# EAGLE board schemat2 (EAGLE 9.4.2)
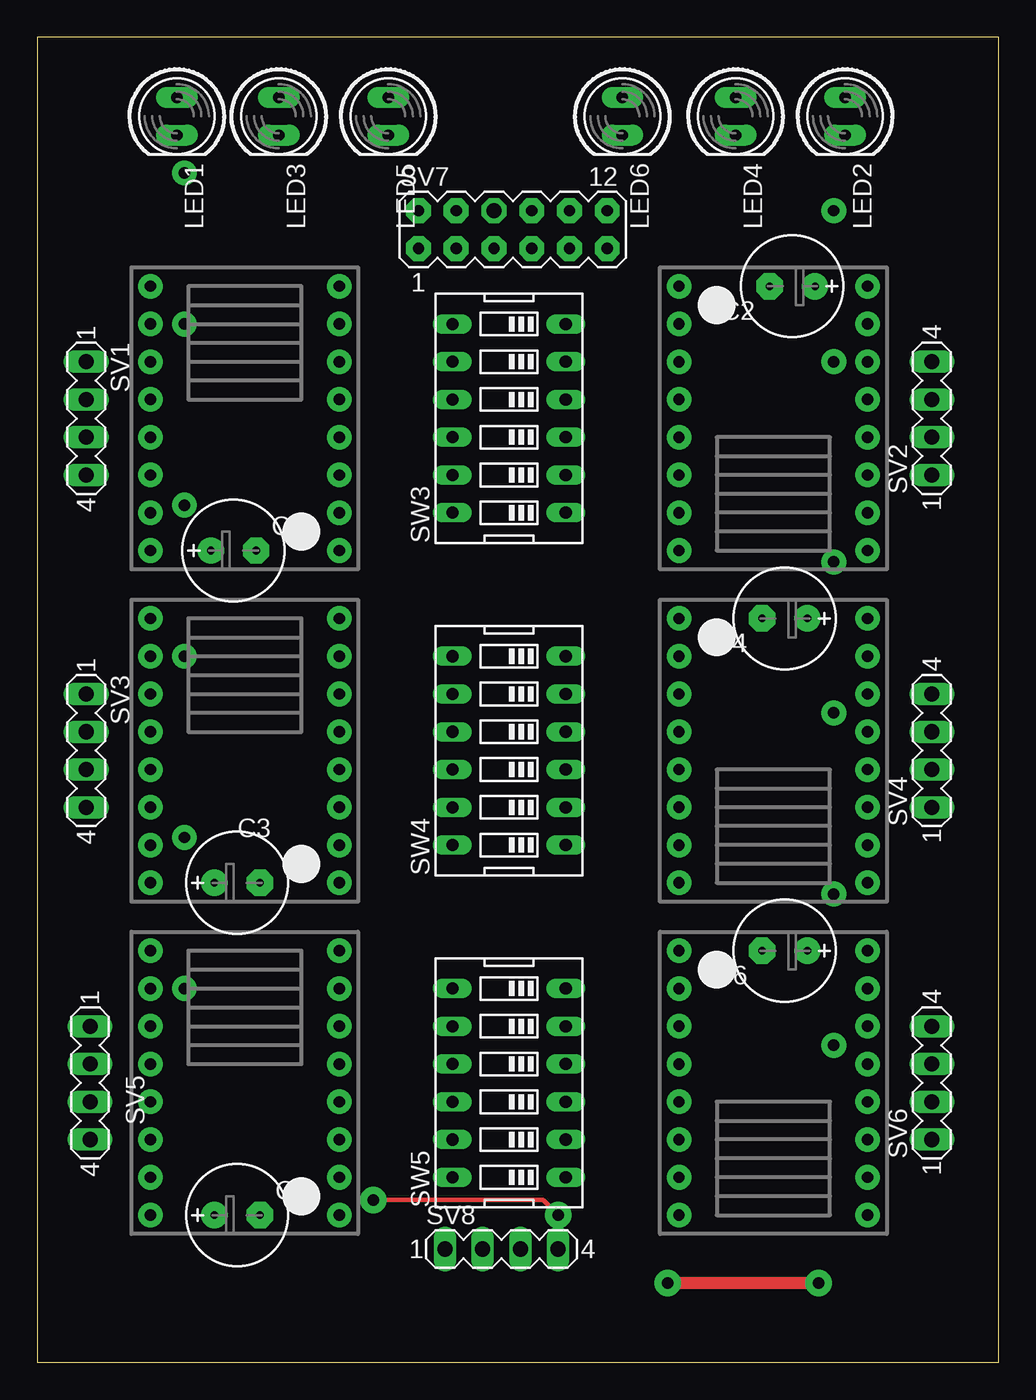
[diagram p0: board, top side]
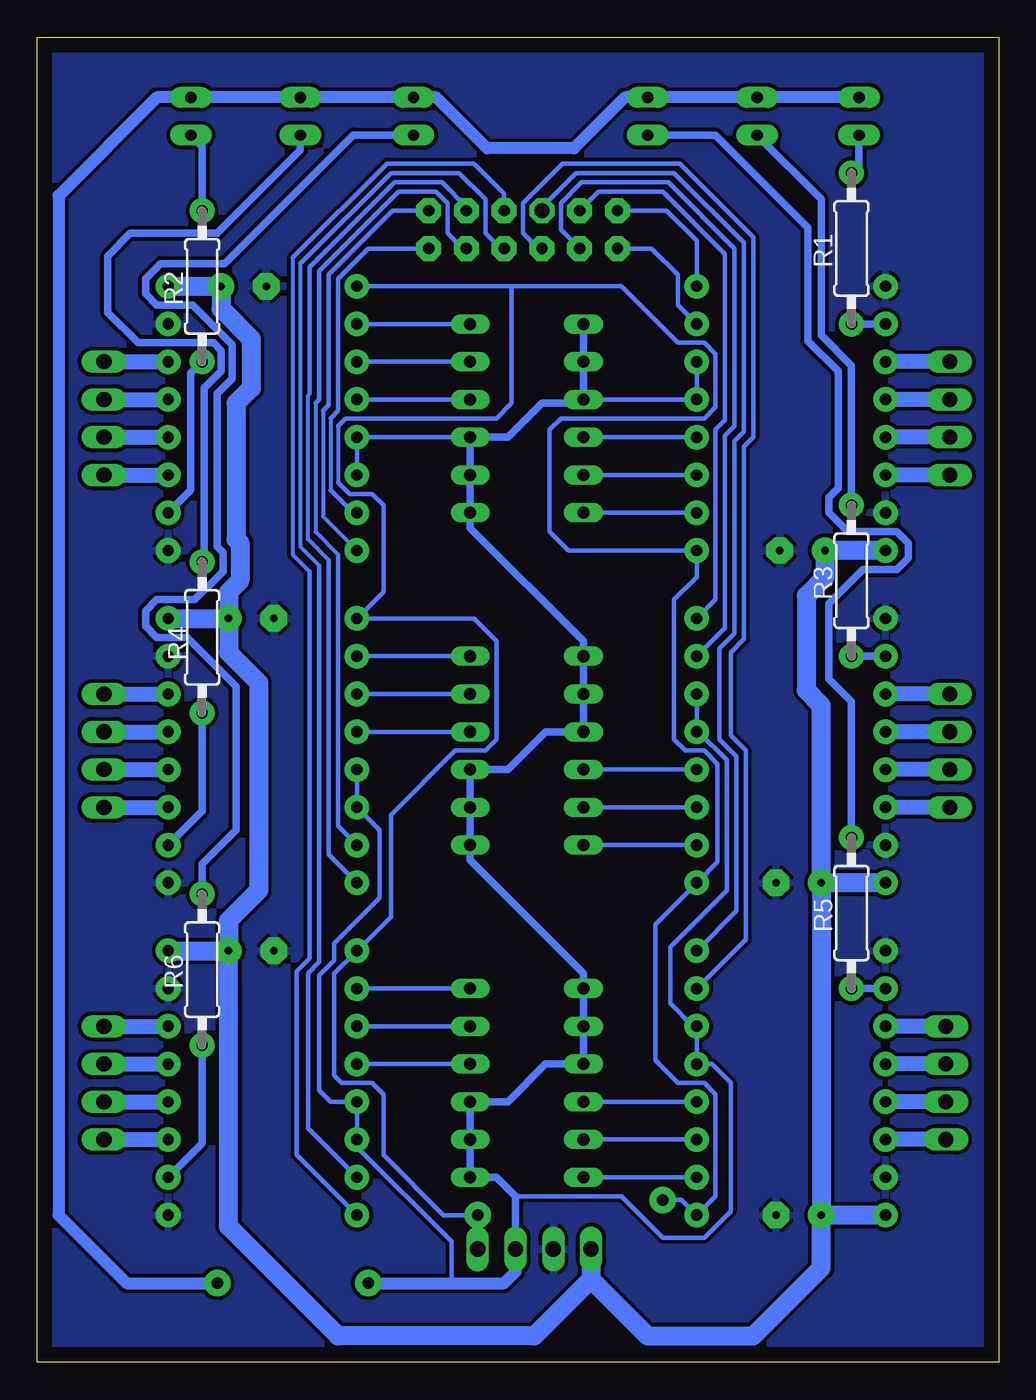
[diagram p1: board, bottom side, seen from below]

Size 64.69 x 89.14 mm. Coordinates in mm from the lower left corner, seen from the top.
Outline: 0,0 64.69,0 64.69,89.14 0,89.14 0,0
Copper layers (1*16): Top 0.035mm / dielectric 1.5mm / Bottom 0.035mm
Design rules "default *": minimum track width 6mil, minimum drill 0.35mm, track to track 8mil, track to pad 8mil, pad to pad 10mil, via to via 10mil, smd to smd 6mil, copper to edge 40mil, drill to drill 6mil, minimum pad ring 10mil, minimum via ring 8mil, stop-mask expansion 4mil, vias tented up to drill 0mil, thermal gap 10mil

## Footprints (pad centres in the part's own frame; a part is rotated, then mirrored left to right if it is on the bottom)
E2,5-7 = drill 0.508 pad 1.778: + -1.524,0 | drill 0.508 pad 1.778 octagon: - 1.524,0
LED5MM = drill 0.762 pad 1.397 long: A -1.27,0; K 1.27,0
0207/10 = drill 0.762 pad 1.676: 1 -5.08,0; 2 5.08,0
MA04-1 = drill 1.016 long: 1 -3.81,0; 2 -1.27,0; 3 1.27,0; 4 3.81,0
MA06-2 = drill 0.762 pad 1.676 octagon: 1 -6.35,-1.27; 2 -6.35,1.27; 3 -3.81,-1.27; 4 -3.81,1.27; 5 -1.27,-1.27; 7 1.27,-1.27; 8 1.27,1.27; 9 3.81,-1.27; 10 3.81,1.27; 11 6.35,-1.27; 12 6.35,1.27 | drill 1.016 pad 1.676 octagon: 6 -1.27,1.27
EDG-06 = drill 0.813 long: 1 -6.35,-3.81; 2 -3.81,-3.81; 3 -1.27,-3.81; 4 1.27,-3.81; 5 3.81,-3.81; 6 6.35,-3.81; 7 6.35,3.81; 8 3.81,3.81; 9 1.27,3.81; 10 -1.27,3.81; 11 -3.81,3.81; 12 -6.35,3.81
DRV8825 = drill 0.762 pad 1.651: 1 -6.35,8.89; 2 -6.35,6.35; 3 -6.35,3.81; 4 -6.35,1.27; 5 -6.35,-1.27; 6 -6.35,-3.81; 7 -6.35,-6.35; 8 -6.35,-8.89; 9 6.35,-8.89; 10 6.35,-6.35; 11 6.35,-3.81; 12 6.35,-1.27; 13 6.35,1.27; 14 6.35,3.81; 15 6.35,6.35; 16 6.35,8.89

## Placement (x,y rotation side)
C1  [E2,5-7]  13.21,54.61 0 top
C2  [E2,5-7]  50.8,72.39 180 top
C3  [E2,5-7]  13.46,32.26 0 top
C4  [E2,5-7]  50.29,50.04 180 top
C5  [E2,5-7]  13.46,9.91 0 top
C6  [E2,5-7]  50.29,27.69 180 top
LED1  [LED5MM]  9.4,83.82 270 top
LED2  [LED5MM]  54.36,83.82 270 top
LED3  [LED5MM]  16.26,83.82 270 top
LED4  [LED5MM]  46.99,83.82 270 top
LED5  [LED5MM]  23.62,83.82 270 top
LED6  [LED5MM]  39.37,83.82 270 top
R1  [0207/10]  9.91,74.93 90 bottom
R2  [0207/10]  53.59,72.39 90 bottom
R3  [0207/10]  9.91,52.58 90 bottom
R4  [0207/10]  53.59,48.77 90 bottom
R5  [0207/10]  9.91,30.23 90 bottom
R6  [0207/10]  53.59,26.42 90 bottom
SV1  [MA04-1]  3.3,63.5 270 top
SV2  [MA04-1]  60.2,63.5 90 top
SV3  [MA04-1]  3.3,41.15 270 top
SV4  [MA04-1]  60.2,41.15 90 top
SV5  [MA04-1]  3.56,18.8 270 top
SV6  [MA04-1]  60.2,18.8 90 top
SV7  [MA06-2]  32,76.2 0 top
SV8  [MA04-1]  31.24,7.62 0 top
SW3  [EDG-06]  31.75,63.5 90 top
SW4  [EDG-06]  31.75,41.15 90 top
SW5  [EDG-06]  31.75,18.8 90 top
U$1  DRV8825  [DRV8825]  13.97,63.5 180 top
U$2  DRV8825  [DRV8825]  49.53,63.5 0 top
U$3  DRV8825  [DRV8825]  13.97,41.15 180 top
U$4  DRV8825  [DRV8825]  49.53,41.15 0 top
U$5  DRV8825  [DRV8825]  13.97,18.8 180 top
U$6  DRV8825  [DRV8825]  49.53,18.8 0 top

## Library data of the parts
C1-C6 = my-rcl; SPICEPREFIX: C
LED1-LED6 = myled
R1-R6 = rcl2; SPICEPREFIX: R
SV1-SV6 SV8 = con-lstb; OC_FARNELL: unknown; OC_NEWARK: unknown
SV7 = my-con-lstb; OC_FARNELL: unknown; OC_NEWARK: unknown
SW3-SW5 = special
U$1-U$6 = robot-driver

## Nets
AX1_DIR: SV7.2 U$1.8
AX1_FLT: R1.1 U$1.10
AX1_M0: SW3.12 U$1.2
AX1_M1: SW3.11 U$1.3
AX1_M2: SW3.10 U$1.4
AX1_STEP: SV7.1 U$1.7
AX2_DIR: SV7.12 U$2.8
AX2_FLT: R2.1 U$2.10
AX2_M0: SW3.6 U$2.2
AX2_M1: SW3.5 U$2.3
AX2_M2: SW3.4 U$2.4
AX2_STEP: SV7.11 U$2.7
AX3_DIR: SV7.4 U$3.8
AX3_FLT: R3.1 U$3.10
AX3_M0: SW4.12 U$3.2
AX3_M1: SW4.11 U$3.3
AX3_M2: SW4.10 U$3.4
AX3_STEP: SV7.3 U$3.7
AX4_DIR: SV7.10 U$4.8
AX4_FLT: R4.1 U$4.10
AX4_M0: SW4.6 U$4.2
AX4_M1: SW4.5 U$4.3
AX4_M2: SW4.4 U$4.4
AX4_STEP: SV7.9 U$4.7
AX5_DIR: SV7.6 U$5.8
AX5_FLT: R5.1 U$5.10
AX5_M0: SW5.12 U$5.2
AX5_M1: SW5.11 U$5.3
AX5_M2: SW5.10 U$5.4
AX5_STEP: SV7.5 U$5.7
AX6_DIR: SV7.8 U$6.8
AX6_FLT: R6.1 U$6.10
AX6_M0: SW5.6 U$6.2
AX6_M1: SW5.5 U$6.3
AX6_M2: SW5.4 U$6.4
AX6_STEP: SV7.7 U$6.7
GND: C1.- C2.- C3.- C4.- C5.- C6.- SV8.2 U$1.9 U$1.15 U$2.9 U$2.15 U$3.9 U$3.15 U$4.9 U$4.15 U$5.9 U$5.15 U$6.9 U$6.15
M_EN: SV8.4 U$1.1 U$2.1 U$3.1 U$4.1 U$5.1 U$6.1
N$1: SV4.1 U$4.11
N$2: LED1.K R1.2
N$3: LED2.K R2.2
N$4: LED3.K R3.2
N$5: LED4.K R4.2
N$6: LED5.K R5.2
N$7: SV4.2 U$4.12
N$8: LED6.K R6.2
N$9: SV5.2 U$5.12
N$10: SV5.1 U$5.11
N$11: SV6.2 U$6.12
N$12: SV6.1 U$6.11
N$13: SV3.2 U$3.12
N$14: SV3.1 U$3.11
N$15: SV2.2 U$2.12
N$16: SV2.1 U$2.11
N$17: SV1.2 U$1.12
N$18: SV1.1 U$1.11
N$21: SV1.4 U$1.14
N$22: SV1.3 U$1.13
N$25: SV2.4 U$2.14
N$26: SV2.3 U$2.13
N$29: SV5.4 U$5.14
N$30: SV5.3 U$5.13
N$33: SV6.4 U$6.14
N$34: SV6.3 U$6.13
N$35: SV4.3 U$4.13
N$36: SV4.4 U$4.14
N$41: SV3.4 U$3.14
N$42: SV3.3 U$3.13
VCC: LED1.A LED2.A LED3.A LED4.A LED5.A LED6.A SV8.3 SW3.1 SW3.2 SW3.3 SW3.7 SW3.8 SW3.9 SW4.1 SW4.2 SW4.3 SW4.7 SW4.8 SW4.9 SW5.1 SW5.2 SW5.3 SW5.7 SW5.8 SW5.9 U$1.5 U$1.6 U$2.5 U$2.6 U$3.5 U$3.6 U$4.5 U$4.6 U$5.5 U$5.6 U$6.5 U$6.6
VMOT: C1.+ C2.+ C3.+ C4.+ C5.+ C6.+ SV8.1 U$1.16 U$2.16 U$3.16 U$4.16 U$5.16 U$6.16

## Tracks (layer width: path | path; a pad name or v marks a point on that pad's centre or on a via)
AX1_DIR
  Bottom 0.305: U$1.8 20.32,75.44 22.35,77.47 SV7.2
AX1_FLT
  Bottom 0.508: U$1.10 R1.1
AX1_M0
  Bottom 0.305: U$1.2 SW3.12
AX1_M1
  Bottom 0.305: U$1.3 SW3.11
AX1_M2
  Bottom 0.305: U$1.4 SW3.10
AX1_STEP
  Bottom 0.305: U$1.7 21.59,71.12 21.59,73.15 23.37,74.93 SV7.1
AX2_DIR
  Bottom 0.254: U$2.8 45.47,56.9 45.47,64.01
  Bottom 0.305: SV7.12 40.77,77.47 45.09,73.15 45.09,64.39 45.47,64.01
AX2_FLT
  Bottom 0.508: R2.1 54.36,66.55 54.36,58.67 U$2.10
AX2_M0
  Bottom 0.305: SW3.6 U$2.2
AX2_M1
  Bottom 0.305: SW3.5 U$2.3
AX2_M2
  Bottom 0.305: SW3.4 U$2.4
AX2_STEP
  Bottom 0.254: 44.96,63.5 44.96,58.67
  Bottom 0.305: SV7.11 42.42,74.93 44.45,72.9 44.45,64.01 44.96,63.5 | 44.96,58.67 43.43,57.15 U$2.7
AX3_DIR
  Bottom 0.305: U$3.8 19.05,51.31 19.05,62.74 18.41,63.37 18.41,74.55 22.61,78.74 26.92,78.74 SV7.4
AX3_FLT
  Bottom 0.508: U$3.10 R3.1
AX3_M0
  Bottom 0.305: U$3.2 SW4.12
AX3_M1
  Bottom 0.305: U$3.3 SW4.11
AX3_M2
  Bottom 0.305: U$3.4 SW4.10
AX3_STEP
  Bottom 0.305: U$3.7 18.41,49.4 18.41,62.36 17.78,62.99 17.78,74.93 22.23,79.38 28.07,79.38 29.46,77.98 29.46,76.2 SV7.3
AX4_DIR
  Bottom 0.254: 45.09,53.98 46.48,55.37 46.48,65.02
  Bottom 0.305: U$4.8 45.09,34.16 45.09,53.98 | SV7.10 35.81,77.72 37.47,79.38 40.64,79.38 46.36,73.66 46.36,65.15 46.48,65.02
AX4_FLT
  Bottom 0.508: U$4.10 53.59,37.08 R4.1
AX4_M0
  Bottom 0.305: U$4.2 SW4.6
AX4_M1
  Bottom 0.305: U$4.3 SW4.5
AX4_M2
  Bottom 0.305: U$4.4 SW4.4
AX4_STEP
  Bottom 0.254: 44.45,54.36 45.97,55.88 45.97,64.52
  Bottom 0.305: U$4.7 44.45,36.07 44.45,54.36 | SV7.9 36.07,74.93 37.08,75.95 37.08,77.98 37.85,78.74 40.39,78.74 45.72,73.41 45.72,64.77 45.97,64.52
AX5_DIR
  Bottom 0.305: SV7.6 30.73,77.72 28.45,80.01 21.84,80.01 17.14,75.31 17.14,62.61 17.78,61.98 17.78,49.02 18.8,48.01 18.8,41.91 17.65,40.77 17.65,30.35 U$5.8
AX5_FLT
  Bottom 0.508: U$5.10 R5.1
AX5_M0
  Bottom 0.305: U$5.2 SW5.12
AX5_M1
  Bottom 0.305: U$5.3 SW5.11
AX5_M2
  Bottom 0.305: U$5.4 SW5.10
AX5_STEP
  Bottom 0.305: U$5.7 17.02,28.45 17.02,41.15 18.03,42.16 18.03,47.75 17.14,48.64 17.14,61.59 16.51,62.23 16.51,75.69 21.46,80.64 29.34,80.64 32,77.98 32,75.95 30.99,74.93 SV7.5
AX6_DIR
  Bottom 0.254: 46.36,53.21 47.5,54.36 47.5,74.29
  Bottom 0.305: U$6.8 47.24,13.97 47.24,26.29 46.36,27.18 46.36,53.21 | 47.5,74.29 41.15,80.64 35.31,80.64 33.27,78.61 SV7.8
AX6_FLT
  Bottom 0.508: U$6.10 53.59,14.73 R6.1
AX6_M0
  Bottom 0.305: SW5.6 U$6.2
AX6_M1
  Bottom 0.305: SW5.5 U$6.3
AX6_M2
  Bottom 0.305: SW5.4 U$6.4
AX6_STEP
  Bottom 0.254: 45.72,53.59 46.99,54.86 46.99,73.91
  Bottom 0.305: 45.72,53.59 45.72,26.92 46.48,26.16 46.48,15.75 U$6.7 | 46.99,73.91 40.89,80.01 36.32,80.01 34.54,78.23 34.54,75.95 33.53,74.93 SV7.7
GND
  pour Bottom (isolate 0.254): 0,89.15 64.77,89.15 64.77,0 0,0
M_EN  (via drill 0.76 pad 1.78)
  Top 0.305: v35.05,9.91 34.04,10.92 v22.61,10.92
  Bottom 0.254: 44.45,62.99 44.45,59.18
  Bottom 0.305: U$2.1 32.77,72.39 | 32.77,72.39 25.4,72.39 21.59,68.58 19.81,68.58 19.05,67.82 19.05,64.26 19.81,63.5 29.46,63.5 30.23,62.74 30.23,55.88 28.96,54.61 U$1.1 20.32,52.83 21.84,51.31 21.84,41.91 21.08,41.15 19.81,41.15 18.92,40.26 18.92,33.66 U$3.1 23.11,29.46 23.11,20.32 21.59,18.8 19.81,18.8 19.05,18.03 19.05,11.18 U$5.1 21.34,10.92 v22.61,10.92 | 32.77,72.39 32.77,64.52 33.78,63.5 43.94,63.5 44.45,62.99 | 44.45,59.18 43.69,58.42 42.16,58.42 41.4,57.66 41.4,51.82 U$4.1 35.31,50.04 33.78,48.51 33.78,41.91 34.54,41.15 36.58,41.15 40.89,36.83 40.89,29.97 U$6.1 44.7,26.16 44.7,19.3 44.2,18.8 42.16,18.8 41.4,18.03 41.4,13.97 37.34,9.91 v35.05,9.91 SV8.4
N$1
  Bottom 1.016: SV4.1 U$4.11
N$2
  Bottom 0.508: LED1.K 9.4,80.52 R1.2
N$3
  Bottom 0.508: LED2.K 53.59,81.79 R2.2
N$4
  Bottom 0.508: R3.2 9.91,67.06 11.94,69.09 11.94,78.23 LED3.K
N$5
  Bottom 0.508: LED4.K 46.99,81.53 52.58,75.95 58.42,75.95 59.94,74.42 59.94,70.61 57.91,68.58 52.83,68.58 52.32,68.07 52.32,66.67 53.47,65.53 53.47,53.98 R4.2
N$6
  Bottom 0.508: R5.2 9.91,44.45 11.43,45.97 11.43,51.05 9.14,53.34 6.86,53.34 6.1,54.1 6.1,55.12 6.86,55.88 10.16,55.88 11.43,57.15 11.43,58.17 10.79,58.8 10.79,66.67 12.83,68.71 12.83,76.33 19.05,82.55 LED5.K
N$7
  Bottom 1.016: SV4.2 U$4.12
N$8
  Bottom 0.508: R6.2 53.59,33.53 51.31,35.81 51.31,45.47 54.61,48.77 56.64,48.77 57.4,49.53 57.4,50.55 56.64,51.31 54.1,51.31 52.2,53.21 52.2,54.48 52.58,54.86 52.58,65.15 51.56,66.17 51.56,68.45 54.23,71.12 56.64,71.12 57.4,71.88 57.4,72.9 56.39,73.91 52.07,73.91 43.43,82.55 LED6.K
N$9
  Bottom 1.016: SV5.2 U$5.12
N$10
  Bottom 1.016: SV5.1 U$5.11
N$11
  Bottom 1.016: SV6.2 U$6.12
N$12
  Bottom 1.016: SV6.1 U$6.11
N$13
  Bottom 1.016: SV3.2 U$3.12
N$14
  Bottom 1.016: SV3.1 U$3.11
N$15
  Bottom 1.016: SV2.2 U$2.12
N$16
  Bottom 1.016: SV2.1 U$2.11
N$17
  Bottom 1.016: SV1.2 U$1.12
N$18
  Bottom 1.016: SV1.1 U$1.11
N$21
  Bottom 1.016: SV1.4 U$1.14
N$22
  Bottom 1.016: SV1.3 U$1.13
N$25
  Bottom 1.016: SV2.4 U$2.14
N$26
  Bottom 1.016: SV2.3 U$2.13
N$29
  Bottom 1.016: SV5.4 U$5.14
N$30
  Bottom 1.016: SV5.3 U$5.13
N$33
  Bottom 1.016: SV6.4 U$6.14
N$34
  Bottom 1.016: SV6.3 U$6.13
N$35
  Bottom 1.016: SV4.3 U$4.13
N$36
  Bottom 1.016: SV4.4 U$4.14
N$41
  Bottom 1.016: SV3.4 U$3.14
N$42
  Bottom 1.016: SV3.3 U$3.13
VCC  (via drill 0.76 pad 1.78)
  Top 0.813: v52.58,5.33 v42.42,5.33
  Bottom 0.305: U$1.6 U$1.5 SW3.9 | U$3.6 U$3.5 20.19,42.42 18.29,40.51 18.29,31.75 22.1,27.94 22.1,24.13 20.57,22.61 U$5.6 U$5.5 19.3,20.07 18.03,18.8 18.03,10.16 19.81,8.38 22.61,8.38 25.4,11.18 32.51,11.18 | U$2.6 U$2.5 SW3.3 | U$4.5 U$4.6 41.66,35.81 41.66,31.24 44.7,28.19 44.7,27.05 45.72,26.04 45.72,18.29 44.96,17.53 U$6.5 U$6.6 43.18,14.48 36.83,8.13 36.83,5.33 | 32.51,6.1 32.51,5.84 33.02,5.33 33.27,5.33
  Bottom 0.508: SW3.7 SW3.8 SW3.9 28.19,64.52 30.73,64.52 33.02,62.23 SW3.3 SW3.2 SW3.1 35.56,56.13 27.94,48.51 SW4.7 SW4.8 SW4.9 30.48,42.42 33.02,39.88 SW4.3 SW4.2 SW4.1 35.56,33.78 27.94,26.16 SW5.7 SW5.8 SW5.9 30.48,20.07 33.02,17.53 SW5.3 SW5.2 SW5.1 33.78,12.45 32.51,11.18 SV8.3
  Bottom 0.813: LED1.A LED3.A LED5.A 25.15,85.09 28.57,81.66 34.42,81.66 37.85,85.09 LED6.A LED4.A LED2.A 56.64,85.09 63.25,78.49 63.25,9.91 58.67,5.33 v52.58,5.33 | v42.42,5.33 36.83,5.33 33.27,5.33 32.51,6.1 SV8.3
VMOT
  Bottom 1.27: U$5.16 C5.+ | U$3.16 C3.+ | U$1.16 C1.+ 11.68,52.83 12.95,51.56 12.95,45.21 11.94,44.2 C3.+ | U$2.16 C2.+ 52.32,70.87 50.29,68.83 50.29,65.53 51.31,64.52 51.31,55.37 51.05,55.12 51.05,52.58 51.82,51.82 C4.+ | U$4.16 C4.+ | U$6.16 C6.+ | C4.+ 51.82,47.75 49.78,45.72 49.78,31.75 51.82,29.72 C6.+ | C5.+ 11.94,6.35 16.51,1.78 23.62,1.78 27.43,5.59 | SV8.1 27.43,5.59 | 27.43,5.59 31.24,1.78 44.45,1.78 51.82,9.14 C6.+ | C3.+ C5.+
